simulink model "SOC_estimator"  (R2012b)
settings: Solver=ode4  StartTime=0.0  StopTime=100  FixedStep=0.001  RelTol=1e-3
undefined symbols (not defined in the file or in its folder): InitialSOC

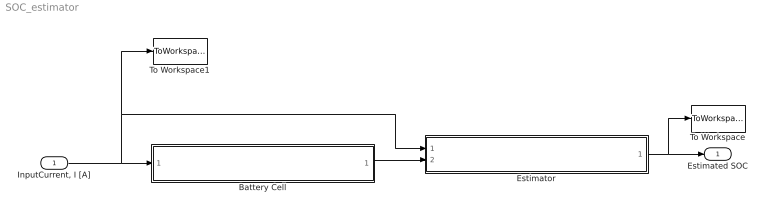
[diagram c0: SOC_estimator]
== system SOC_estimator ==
  "InputCurrent, I [A]" : Inport
  Battery Cell : Subsystem
  Estimator : Subsystem
  To Workspace : ToWorkspace  VariableName=EstSOC  SampleTime=-1  SaveFormat=Structure With Time
  To Workspace1 : ToWorkspace  VariableName=InputCurrent  SampleTime=-1  SaveFormat=Structure With Time
  Estimated SOC : Outport
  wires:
  Battery Cell/1("OutputVoltage, V_b [v]") -> Estimator/2("Voltage, V_b [v]")
  "InputCurrent, I [A]"/1 -> To Workspace1/1, Estimator/1("Current, I_b [A]"), Battery Cell/1("InputCurrent, I_b [A]")
  Estimator/1(Estimated SOC) -> To Workspace/1, Estimated SOC/1

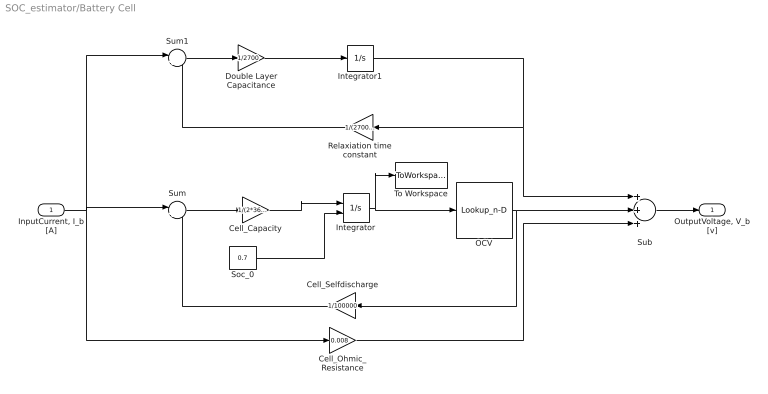
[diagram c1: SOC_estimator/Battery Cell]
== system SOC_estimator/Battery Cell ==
  "InputCurrent, I_b [A]" : Inport
  Cell_Capacity : Gain  Gain=1/(2*3600)
  Cell_Ohmic_Resistance : Gain  Gain=0.008
  Cell_Selfdischarge : Gain  Gain=1/100000
  Double Layer Capacitance : Gain  Gain=1/2700
  Integrator : Integrator  InitialConditionSource=external  InitialCondition=InitialSOC
  Integrator1 : Integrator
  OCV : Lookup_n-D  NumberOfTableDimensions=1  BreakpointsForDimension1=[0 0.1 0.2 0.3 0.4 0.5 0.6 0.7 0.8 0.9 1]  Table=[2.25 3.2 3.25 3.25 3.3 3.3 3.3 3.35 3.35 3.35 3.75]  RndMeth=Simplest
  Relaxiation time constant : Gain  Gain=1/(2700*0.011)
  Soc_0 : Constant  Value=0.7
  Sub : Sum  Inputs=+++
  Sum : Sum  Inputs=|+-
  Sum1 : Sum  Inputs=|+-
  To Workspace : ToWorkspace  VariableName=SOC  SampleTime=-1  SaveFormat=Structure With Time
  "OutputVoltage, V_b [v]" : Outport
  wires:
  Integrator/1 -> To Workspace/1, OCV/1
  OCV/1 -> Cell_Selfdischarge/1, Sub/2
  "InputCurrent, I_b [A]"/1 -> Sum1/1, Cell_Ohmic_Resistance/1, Sum/1
  Cell_Capacity/1 -> Integrator/1
  Cell_Selfdischarge/1 -> Sum/2
  Integrator1/1 -> Relaxiation time constant/1, Sub/1
  Relaxiation time constant/1 -> Sum1/2
  Cell_Ohmic_Resistance/1 -> Sub/3
  Sub/1 -> "OutputVoltage, V_b [v]"/1
  Sum/1 -> Cell_Capacity/1
  Double Layer Capacitance/1 -> Integrator1/1
  Sum1/1 -> Double Layer Capacitance/1
  Soc_0/1 -> Integrator/2

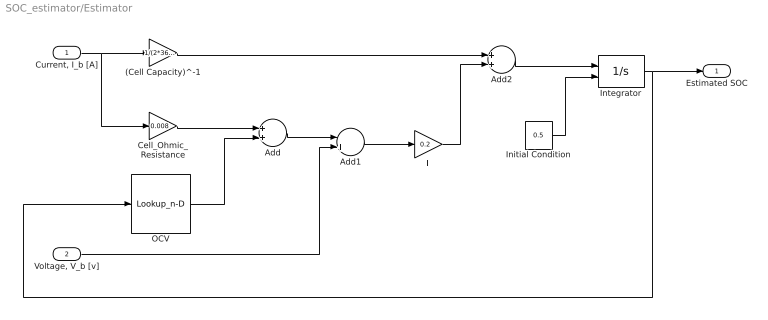
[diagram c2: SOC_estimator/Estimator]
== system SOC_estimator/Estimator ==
  "Current, I_b [A]" : Inport
  "Voltage, V_b [v]" : Inport  Port=2
  (Cell Capacity)^-1 : Gain  Gain=1/(2*3600)
  Add : Sum
  Add1 : Sum  Inputs=-+
  Add2 : Sum
  Cell_Ohmic_Resistance : Gain  Gain=0.008
  Initial Condition : Constant  Value=0.5
  Integrator : Integrator  InitialConditionSource=external
  L : Gain  Gain=0.2
  OCV : Lookup_n-D  NumberOfTableDimensions=1  BreakpointsForDimension1=[0 0.1 0.2 0.3 0.4 0.5 0.6 0.7 0.8 0.9 1]  Table=[2.25 3.2 3.25 3.25 3.3 3.3 3.3 3.35 3.35 3.35 3.75]  RndMeth=Simplest
  Estimated SOC : Outport
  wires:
  "Current, I_b [A]"/1 -> Cell_Ohmic_Resistance/1, (Cell Capacity)^-1/1
  Cell_Ohmic_Resistance/1 -> Add/1
  OCV/1 -> Add/2
  Add/1 -> Add1/1
  "Voltage, V_b [v]"/1 -> Add1/2
  Add1/1 -> L/1
  (Cell Capacity)^-1/1 -> Add2/1
  L/1 -> Add2/2
  Add2/1 -> Integrator/1
  Initial Condition/1 -> Integrator/2
  Integrator/1 -> Estimated SOC/1, OCV/1
